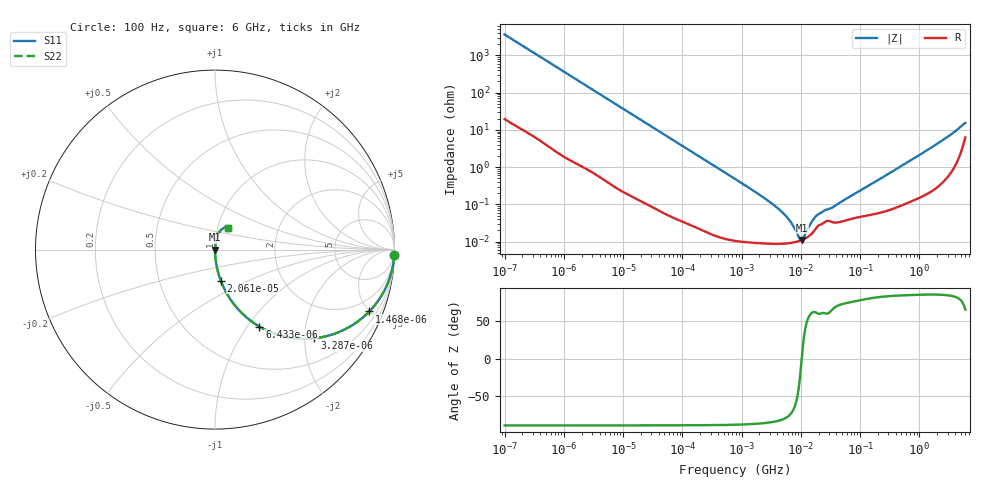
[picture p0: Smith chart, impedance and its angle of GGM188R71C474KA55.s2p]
!Murata Part Number: GGM188R71C474KA55
!These Parameters are Measured in Series Mode Connection
!Data Generated on Mar 13, 2026
!  o--ll--o
!Port1  Port2
!  o------o
!Operation Temp=25[degC], DC Bias Voltage=0[V]
!Freq. Start=100[Hz] Stop=6[GHz] 401[Steps]
# Hz S RI R 50
!Freq.(Hz) S11(Real) S11(Imag) S21(Real) S21(Imag) S12(Real) S12(Imag) S22(Real) S22(Imag)
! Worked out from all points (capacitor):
!   401 points, 100 Hz to 6 GHz, reference 50 ohm
!   read as one part in series: C = 439 nF near 109 Hz
!   lowest |Z| = 11 mohm at 10.4 MHz (marker M1)
!   series resonance near 10.34 MHz, so ESL is about 540 pH
!   S11 on the Smith chart (normalised r, x): 100 Hz: 1, -72; 1.468 kHz: 1.03, -4.98; 3.287 kHz: 1.01, -2.23; 6.433 kHz: 1.01, -1.14; 20.61 kHz: 1.00, -0.36; 6 GHz: 1.12, +0.28
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100  0.9991 -0.0276  0.000909 0.0276  0.000909 0.0276  0.9991 -0.0276
458  0.9838 -0.1237  0.0162 0.1237  0.0162 0.1237  0.9838 -0.1237
1468  0.8598 -0.3445  0.1402 0.3445  0.1402 0.3445  0.8598 -0.3445
2008  0.7672 -0.4198  0.2328 0.4198  0.2328 0.4198  0.7672 -0.4198
3287  0.5542 -0.4941  0.4458 0.4941  0.4458 0.4941  0.5542 -0.4941
6433  0.2474 -0.4286  0.7526 0.4286  0.7526 0.4286  0.2474 -0.4286
11009  0.102 -0.2997  0.898 0.2997  0.898 0.2997  0.102 -0.2997
20606  0.0322 -0.1731  0.9678 0.1731  0.9678 0.1731  0.0322 -0.1731
40335  0.009 -0.0909  0.991 0.0909  0.991 0.0909  0.009 -0.0909
774597  0.000127 -0.00481  0.9999 0.00481  0.9999 0.00481  0.000127 -0.00481
4440638  8.71e-05 -0.000695  0.9999 0.000695  0.9999 0.000695  8.71e-05 -0.000695
6353432  9.05e-05 -0.000371  0.9999 0.000371  0.9999 0.000371  9.05e-05 -0.000371
9506416  0.000105 -6.21e-05  0.9999 6.21e-05  0.9999 6.21e-05  0.000105 -6.21e-05
1.039699e7  0.00011 3.9e-06  0.9999 -3.9e-06  0.9999 -3.9e-06  0.00011 3.9e-06
1.137099e7  0.000117 7.01e-05  0.9999 -7.01e-05  0.9999 -7.01e-05  0.000117 7.01e-05
1.555665e7  0.000167 0.000312  0.9998 -0.000312  0.9998 -0.000312  0.000167 0.000312
1.86079e7  0.000241 0.000443  0.9998 -0.000443  0.9998 -0.000443  0.000241 0.000443
2.327686e7  0.000303 0.000556  0.9997 -0.000556  0.9997 -0.000556  0.000303 0.000556
3.482834e7  0.000329 0.000769  0.9997 -0.000769  0.9997 -0.000769  0.000329 0.000769
3.124326e8  0.000746 0.00677  0.9993 -0.00677  0.9993 -0.00677  0.000746 0.00677
3.205649e9  0.0108 0.0682  0.9892 -0.0682  0.9892 -0.0682  0.0108 0.0682
6e9  0.0746 0.1215  0.9254 -0.1215  0.9254 -0.1215  0.0746 0.1215
